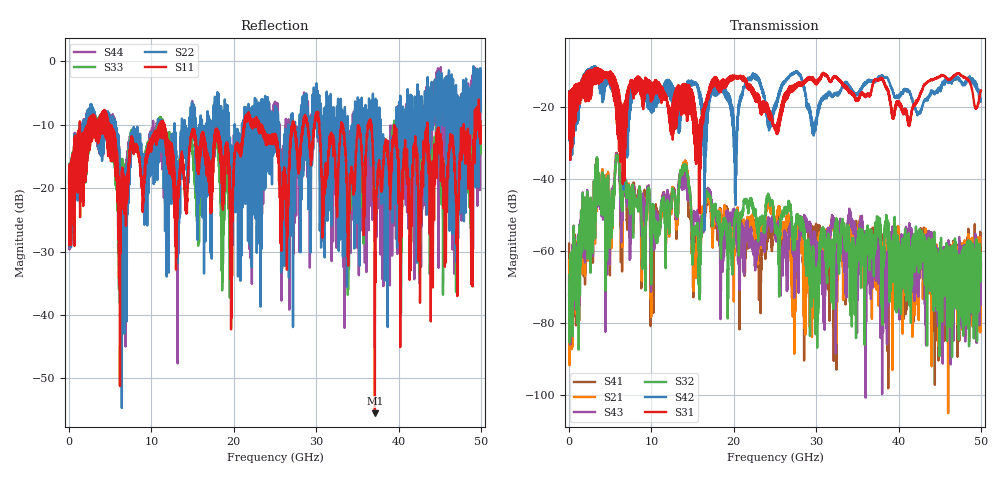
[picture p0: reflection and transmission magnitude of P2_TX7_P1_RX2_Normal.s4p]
!Keysight Technologies,N5225B,MY57041031,A.13.20.10
!Date: Friday, May 31, 2019 11:16:51
!Correction: S11(Full 4 Port(1,2,3,4))
!S12(Full 4 Port(1,2,3,4))
!S13(Full 4 Port(1,2,3,4))
!S14(Full 4 Port(1,2,3,4))
!S21(Full 4 Port(1,2,3,4))
!S22(Full 4 Port(1,2,3,4))
!S23(Full 4 Port(1,2,3,4))
!S24(Full 4 Port(1,2,3,4))
!S31(Full 4 Port(1,2,3,4))
!S32(Full 4 Port(1,2,3,4))
!S33(Full 4 Port(1,2,3,4))
!S34(Full 4 Port(1,2,3,4))
!S41(Full 4 Port(1,2,3,4))
!S42(Full 4 Port(1,2,3,4))
!S43(Full 4 Port(1,2,3,4))
!S44(Full 4 Port(1,2,3,4))
!S4P File: Measurements: <S11,S12,S13,S14>,
!<S21,S22,S23,S24>,
!<S31,S32,S33,S34>,
!<S41,S42,S43,S44>:
# Hz S  dB  R 50.0
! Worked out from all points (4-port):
!   5000 points, 10 MHz to 50 GHz, reference 50 ohm
!   strongest paths, dB at 10 MHz, 12.51 GHz, 25.01 GHz, 37.51 GHz, 50 GHz:
!     S31: -19.6, -21.0, -25.9, -12.8, -15.5
!     S42: -19.4, -16.4, -19.4, -12.3, -17.8
!     S32: -72.2, -43.6, -54.1, -51.4, -67.8
!     S43: -67.3, -44.2, -53.7, -60.7, -64.1
!     S21: -62.5, -43.4, -52.0, -61.0, -64.1
!     S41: -57.9, -43.4, -53.0, -61.1, -63.7
!   lowest |S11| = -55.5 dB at 37.13 GHz (marker M1), VSWR 1.00, Z = 50.2 + j0.0108 ohm
!   |S11| at or under -10 dB: 4.96 GHz to 11.03 GHz (6.066 GHz wide, 75.9 % of centre); 11.57 GHz to 21.26 GHz (9.684 GHz wide, 59 % of centre); 36.74 GHz to 43.5 GHz (6.762 GHz wide, 16.9 % of centre)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
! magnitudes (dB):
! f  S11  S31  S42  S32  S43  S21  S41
! 10 MHz  -20.2  -19.6  -19.4  -72.2  -67.3  -62.5  -57.9
! 5.85 GHz  -15.6  -17.4  -17.3  -33.8  -33.7  -33.6  -33.5
! 9.07 GHz  -20.8  -13.9  -16.6  -59.0  -46.1  -46.7  -46.1
! 14.04 GHz  -19.3  -16.2  -15.2  -36.8  -39.5  -35.8  -38.1
! 15.21 GHz  -10.9  -27.9  -13.8  -53.5  -50.4  -64.7  -56.3
! 37.13 GHz  -55.5  -12.5  -12.7  -58.9  -60.1  -67.4  -54.2
! 50 GHz  -11.0  -15.5  -17.8  -67.8  -64.1  -64.1  -63.7
